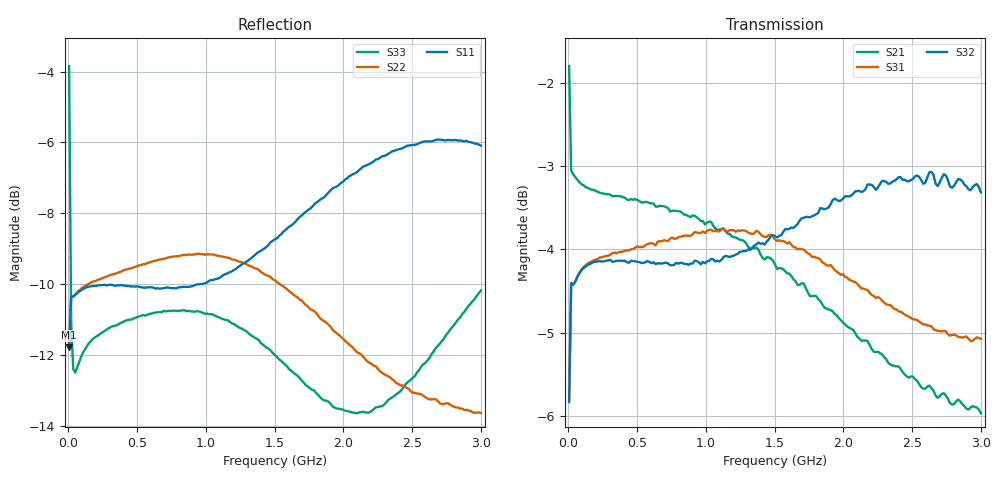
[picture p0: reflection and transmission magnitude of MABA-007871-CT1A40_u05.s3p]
#	MHz	S	RI	R	50
!FREQ	R1	I1	R2	I2	R3	I3
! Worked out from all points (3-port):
!   201 points, 5 MHz to 3 GHz, reference 50 ohm
!   strongest paths, dB at 5 MHz, 753.8 MHz, 1.502 GHz, 2.251 GHz, 3 GHz:
!     S32: -5.8, -4.2, -3.8, -3.3, -3.3
!     S31: -5.8, -3.9, -3.9, -4.6, -5.1
!     S21: -1.8, -3.5, -4.2, -5.2, -6.0
!   lowest |S11| = -11.8 dB at 5 MHz (marker M1), VSWR 1.69, Z = 71.4 + j23.6 ohm
!   |S11| at or under -10 dB: start of sweep to 951.5 MHz
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5  0.2063 0.1542  0.7949 -0.1602  -0.4125 -0.3037
   0.7966 -0.161  0.2037 0.1566  0.4111 0.3051
   -0.4125 -0.3037  0.4055 0.3107  -0.1795 0.6165
19.975  0.3011 0.0397  0.7009 -0.065  -0.5953 -0.085
        0.7008 -0.0652  0.3 0.0501  0.5941 0.095
        -0.5953 -0.085  0.5949 0.0941  0.1943 0.2001
94.85  0.3087 -0.0327  0.6842 -0.0898  -0.6127 0.0324
       0.6846 -0.0898  0.3115 0.0168  0.6127 0.0176
       -0.6127 0.0324  0.6127 0.0175  0.2392 0.0743
828.625  0.00916 -0.3133  0.3994 -0.5339  -0.3792 0.5188
         0.4006 -0.5288  0.3422 -0.06  0.6073 -0.1203
         -0.3792 0.5188  0.6071 -0.1219  0.2899 -0.0165
1158.075  -0.2055 -0.2551  0.159 -0.6273  -0.1558 0.6276
          0.1691 -0.6223  0.3263 -0.1112  0.6034 -0.1648
          -0.1558 0.6276  0.6017 -0.168  0.2773 -0.0477
1502.5  -0.3614 -0.058  -0.1098 -0.6042  0.0981 0.6321
        -0.0946 -0.6106  0.281 -0.1533  0.6057 -0.2228
        0.0981 0.6321  0.6022 -0.2243  0.2435 -0.0617
1921.8  -0.3462 0.2582  -0.3665 -0.4278  0.3493 0.5067
        -0.363 -0.4514  0.2168 -0.1653  0.6002 -0.3176
        0.3493 0.5067  0.5971 -0.3157  0.2091 -0.0382
2356.075  -0.1018 0.4763  -0.4872 -0.1652  0.4942 0.3083
          -0.5057 -0.1818  0.1747 -0.1528  0.5549 -0.4342
          0.4942 0.3083  0.5487 -0.4229  0.2189 0.00467
2685.525  0.1403 0.4862  -0.4884 0.0384  0.5423 0.1543
          -0.5124 0.0406  0.1588 -0.1471  0.485 -0.5141
          0.5423 0.1543  0.4772 -0.4965  0.2575 0.0245
3000  0.3287 0.3715  -0.4319 0.2201  0.5574 0.00684
      -0.443 0.2383  0.1432 -0.151  0.3935 -0.5762
      0.5574 0.00684  0.3942 -0.5575  0.3092 0.0194
